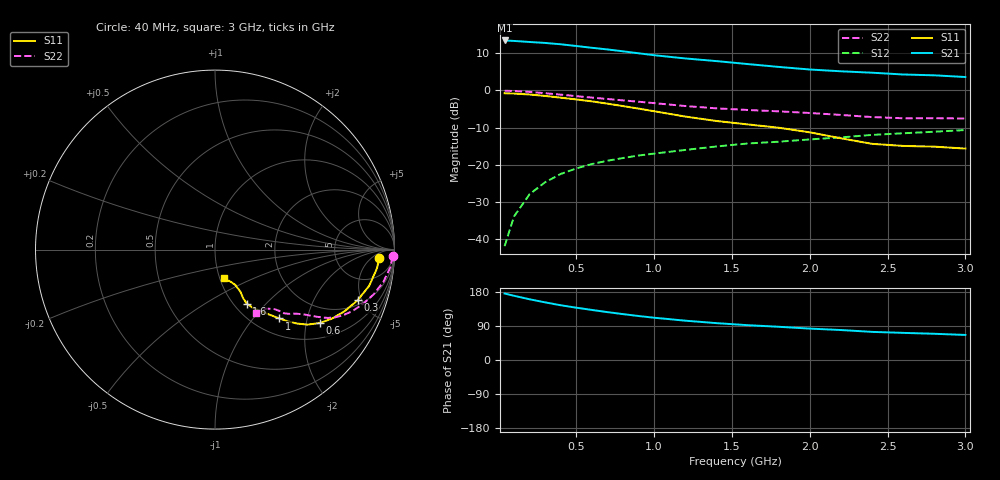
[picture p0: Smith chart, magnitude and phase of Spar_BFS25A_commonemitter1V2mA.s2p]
! Filename:  BFS25AE.S2P  Version:  4.0
! NXP part #: BFS25A  Date: Jun 1994
! Bias condition: Vce=1V, Ic=2mA
#  MHz  S  MA  R  50
! Freq  S11  S21  S12  S22  !GUM [dB]
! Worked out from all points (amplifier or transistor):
!   21 points, 40 MHz to 3 GHz, reference 50 ohm
!   highest |S21| = 13.5 dB at 40 MHz (marker M1)
!   |S21| within 3 dB of that: start of sweep to 814.6 MHz
!   unconditionally stable (mu >= 1): 1.641 GHz to end of sweep
!   at 300 MHz: K = 0.32, MSG = 18.8 dB, |S12| = -24.7 dB
!   at 1 GHz: K = 0.78, MSG = 13.3 dB, |S12| = -17.0 dB
!   at 3 GHz: K = 1.15, MAG = 4.8 dB, |S12| = -10.7 dB
!   lowest NFmin = 2.50 dB at 500 MHz
!   S11 on the Smith chart (normalised r, x): 40 MHz: 18, -10; 300 MHz: 2.37, -4.62; 600 MHz: 1.44, -2.40; 1 GHz: 1.30, -1.37; 1.6 GHz: 1.14, -0.78; 3 GHz: 1.05, -0.34
40  0.917 -2.8  4.71 175.4  0.008 87.9  0.99 -2.2
100  0.908 -6.7  4.641 169.5  0.02 83.8  0.983 -5.6
200  0.882 -13.3  4.493 160.3  0.04 78.7  0.955 -10.9
300  0.843 -19.6  4.361 152.1  0.058 74.6  0.918 -15.8
400  0.799 -25.5  4.185 144.5  0.075 71.5  0.878 -20.2
500  0.757 -30.5  3.967 138.1  0.089 68.7  0.838 -24.2
600  0.713 -35.0  3.753 132.1  0.102 66.7  0.801 -27.2
700  0.664 -39.0  3.567 126.4  0.113 65.1  0.767 -29.5
800  0.616 -42.0  3.364 121.1  0.123 63.9  0.735 -31.2
900  0.57 -44.6  3.167 116.1  0.133 62.6  0.705 -32.4
1000  0.525 -46.9  2.981 111.6  0.141 61.6  0.675 -33.6
1200  0.445 -52.1  2.697 103.8  0.158 59.6  0.617 -35.9
1400  0.388 -56.9  2.485 97.3  0.176 58.8  0.574 -38.4
1600  0.349 -59.6  2.267 91.9  0.193 57.6  0.546 -41.0
1800  0.315 -59.9  2.074 87.7  0.204 57.5  0.523 -42.7
2000  0.273 -58.9  1.914 82.9  0.219 56.9  0.497 -43.5
2200  0.227 -60.1  1.811 79.1  0.233 56.4  0.468 -45.1
2400  0.191 -65.5  1.733 74.2  0.252 55.3  0.438 -48.7
2600  0.179 -73.6  1.64 71.6  0.265 54.2  0.422 -53.1
2800  0.175 -76.5  1.598 69.2  0.278 54.7  0.423 -56.1
3000  0.165 -72.6  1.516 66.1  0.293 54.1  0.419 -57.4
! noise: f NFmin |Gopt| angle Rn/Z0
500  2.5  0.746  4  1.9
1000  2.6  0.716  10  1.9
2000  3.1  0.647  27  1.3
